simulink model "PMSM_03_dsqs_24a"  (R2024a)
settings: Solver=ode45  StartTime=0.0  StopTime=0.1  RelTol=1e-3  EnableMultiTasking=on
undefined symbols (not defined in the file): by, established, Flux, linkage, magnets, V
libraries: spsControlledVoltageSourceLib x3, spsCurrentMeasurementLib x3, spsPermanentMagnetSynchronousMachineLib x1, spspowerguiLib x1

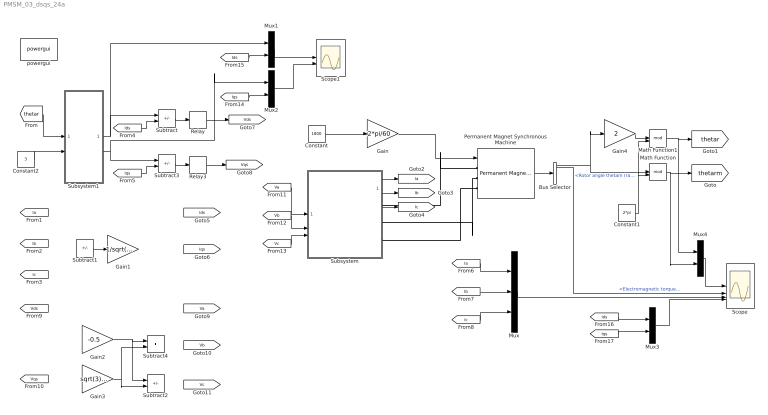
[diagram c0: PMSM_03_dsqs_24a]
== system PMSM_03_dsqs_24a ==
  Bus Selector : BusSelector  OutputSignals=Rotor angle thetam (rad),Electromagnetic torque Te (N*m)
  Constant : Constant  Value=1800
  Constant1 : Constant  Value=2*pi
  Constant2 : Constant  Value=3
  Gain : Gain  Gain=2*pi/60
  Gain1 : Gain  Gain=1/sqrt(3)
  Gain2 : Gain  Gain=-0.5
  Gain3 : Gain  Gain=sqrt(3)/2
  Gain4 : Gain  Gain=2
  Math Function : Math  Operator=mod  SignedPower=on
  Math Function1 : Math  Operator=mod  SignedPower=on
  Mux : Mux  Inputs=3
  Mux{1..4} (4 alike) : Mux  Inputs=2
  Permanent Magnet Synchronous Machine : spsPermanentMagnetSynchronousMachineLib/Permanent Magnet Synchronous Machine  NbPhases=3  FluxDistribution=Sinusoidal  RotorType=Round  MechanicalLoad=Speed w  PresetModel=No  ShowDetailedParameters=on  MeasurementBus=off  Resistance=0.423  Inductance=8.5e-3  dqInductances=[8.5e-3,8.5e-3]  La=0.00476  MachineConstant=Flux linkage established by magnets (V.s)  Flux=0.422  VoltageCst=153.0847  TorqueCst=1.266  Flat=120  Mechanical=[0.03 0.04 4 0]  PolePairs=2  InitialConditions=[0,0, 0,0]  InitialConditions5ph=[0 0 0 0 0 0]  RefAngle=Aligned with phase A axis (original Park)  IterativeDiscreteModel=Trapezoidal non iterative  TsBlock=-1  TsPowergui=0
  Relay : Relay  OnSwitchValue=0.2  OffSwitchValue=-0.2  OffOutputValue=-1
  Relay3 : Relay  OnSwitchValue=0.2  OffSwitchValue=-0.2  OffOutputValue=-1
  Scope : Scope  NumInputPorts=4
  Scope1 : Scope  NumInputPorts=2
  Subsystem : Subsystem
  Subsystem1 : Subsystem
  Subtract{,1..3} (4 alike) : Sum  Inputs=+-
  Subtract4 : Sum
  powergui : spspowerguiLib/powergui  Priority=1  SimulationMode=Continuous  SampleTime=50e-6  frequency=60  Iterations=50  frequencyindice=0  Pbase=100e6  ErrMax=1e-4  UnitsV=kV  UnitsW=MW  buscounter=0  FunctionMessages=off  echomessages=off  EnableUseOfTLC=off  CurrentSourceSwitches=off  DisableSnubberDevices=on  DisableRonSwitches=on  DisableVfSwitches=on  DisplayEquations=off  AutomaticDiscreteSolvers=off  SolverType=Tustin  Interpol=off  ExternalGateDelay=off  methode=off  Ts=0  x0status=blocks  SPID=on  SwTol=0  HookPort=off  NonlinearTolerance=1e-4  nMaxIteration=100  ContinueOnMaxIteration=off  RestoreLinks=warning  ResistiveCurrentMeasurement=off  Frange=[0:2:500]  Ylog=off  Xlog=on  ShowGrid=off  save=off  variable=ZData  structure=0  ZoomFFT=off  StartTime=0.0  cycles=1  DisplayStyle=1  fundamental=60  FreqAxis=off  MaxFrequency=1000  frequencyindicesteady=1  RmsSteady=1  display=off
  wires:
  Gain/1 -> Permanent Magnet Synchronous Machine/1
  Constant/1 -> Gain/1
  Subtract/1 -> Relay/1
  Permanent Magnet Synchronous Machine/1 -> Bus Selector/1
  Mux/1 -> Scope/3
  Bus Selector/2 -> Scope/2  "<Electromagnetic torque Te (N*m)>"
  Bus Selector/1 -> Gain4/1, Math Function/1  "<Rotor angle thetam (rad)>"
  Constant1/1 -> Math Function1/2, Math Function/2
  Math Function/1 -> Mux4/2, [thetarm]
  Gain4/1 -> Math Function1/1
  Math Function1/1 -> Mux4/1, [thetar]
  [thetar] -> Subsystem1/1(In1)
  Constant2/1 -> Subsystem1/2(In2)
  Subtract3/1 -> Relay3/1
  Subsystem1/1(Out1) -> Mux1/1, Subtract/1
  Subsystem1/2(Out2) -> Mux2/1, Subtract3/1
  Subsystem/1(Out1) -> [Ia]
  Subsystem/2(Out2) -> [Ib]
  Subsystem/3(Out3) -> [Ic]
  [Ids] -> Subtract/2
  [Iqs] -> Subtract3/2
  [Ia] -> Mux/1
  [Ib] -> Mux/2
  [Ic] -> Mux/3
  Relay/1 -> [Vds]
  Relay3/1 -> [Vqs]
  [Vc] -> Subsystem/3(In3)
  [Vb] -> Subsystem/2(In2)
  [Va] -> Subsystem/1(In1)
  Mux2/1 -> Scope1/2
  Mux1/1 -> Scope1/1
  [Ids] -> Mux1/2
  [Iqs] -> Mux2/2
  Mux3/1 -> Scope/4
  [Ids] -> Mux3/1
  [Iqs] -> Mux3/2
  Mux4/1 -> Scope/1
  Subtract1/1 -> Gain1/1
  Gain2/1 -> Subtract2/1, Subtract4/1
  Gain3/1 -> Subtract2/2, Subtract4/2
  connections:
  Subsystem/RConn1 -- Permanent Magnet Synchronous Machine/LConn1
  Permanent Magnet Synchronous Machine/LConn2 -- Subsystem/RConn2
  Subsystem/RConn3 -- Permanent Magnet Synchronous Machine/LConn3

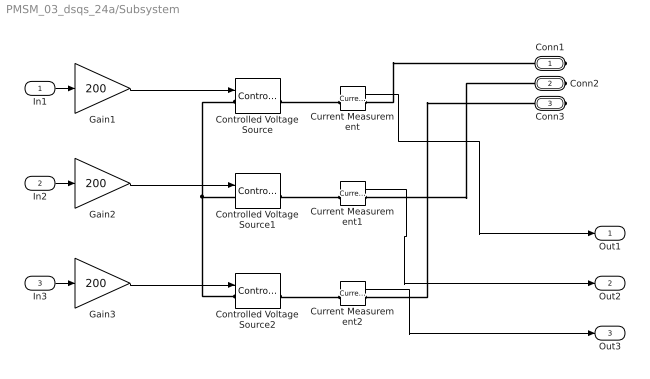
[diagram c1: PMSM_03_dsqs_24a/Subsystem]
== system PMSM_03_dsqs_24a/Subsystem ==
  In1 : Inport
  In2 : Inport  Port=2
  In3 : Inport  Port=3
  Controlled Voltage Source : spsControlledVoltageSourceLib/Controlled Voltage Source  Initialize=on  Source_Type=AC  Amplitude=0  Phase=0  Frequency=0  Measurements=None
  Controlled Voltage Source1 : spsControlledVoltageSourceLib/Controlled Voltage Source  Initialize=on  Source_Type=AC  Amplitude=0  Phase=0  Frequency=0  Measurements=None
  Controlled Voltage Source2 : spsControlledVoltageSourceLib/Controlled Voltage Source  Initialize=on  Source_Type=AC  Amplitude=0  Phase=0  Frequency=0  Measurements=None
  Current Measurement : spsCurrentMeasurementLib/Current Measurement  PhasorSimulation=off  OutputType=Complex  PSBequivalent=0
  Current Measurement1 : spsCurrentMeasurementLib/Current Measurement  PhasorSimulation=off  OutputType=Complex  PSBequivalent=0
  Current Measurement2 : spsCurrentMeasurementLib/Current Measurement  PhasorSimulation=off  OutputType=Complex  PSBequivalent=0
  Gain1 : Gain  Gain=200
  Gain2 : Gain  Gain=200
  Gain3 : Gain  Gain=200
  Conn1 : PMIOPort  Side=Right
  Conn2 : PMIOPort  Port=2  Side=Right
  Conn3 : PMIOPort  Port=3  Side=Right
  Out1 : Outport
  Out2 : Outport  Port=2
  Out3 : Outport  Port=3
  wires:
  In1/1 -> Gain1/1
  In2/1 -> Gain2/1
  In3/1 -> Gain3/1
  Current Measurement1/1 -> Out2/1
  Gain3/1 -> Controlled Voltage Source2/1
  Gain2/1 -> Controlled Voltage Source1/1
  Gain1/1 -> Controlled Voltage Source/1
  Current Measurement2/1 -> Out3/1
  Current Measurement/1 -> Out1/1
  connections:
  Current Measurement/RConn1 -- Conn1/RConn1
  Controlled Voltage Source/LConn1 -- Controlled Voltage Source1/LConn1 -- Controlled Voltage Source2/LConn1
  Controlled Voltage Source/RConn1 -- Current Measurement/LConn1
  Conn2/RConn1 -- Current Measurement1/RConn1
  Current Measurement2/RConn1 -- Conn3/RConn1
  Controlled Voltage Source1/RConn1 -- Current Measurement1/LConn1
  Controlled Voltage Source2/RConn1 -- Current Measurement2/LConn1

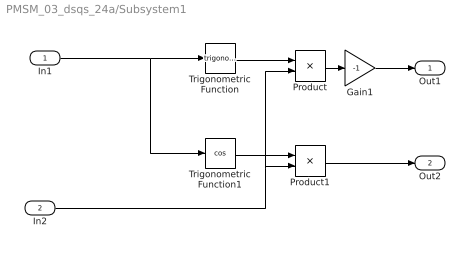
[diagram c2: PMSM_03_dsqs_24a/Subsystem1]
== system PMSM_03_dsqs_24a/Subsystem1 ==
  In1 : Inport
  In2 : Inport  Port=2
  Gain1 : Gain  Gain=-1
  Product : Product
  Product1 : Product
  Trigonometric Function : Trigonometry
  Trigonometric Function1 : Trigonometry  Operator=cos
  Out1 : Outport
  Out2 : Outport  Port=2
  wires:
  Trigonometric Function1/1 -> Product1/1
  Product/1 -> Gain1/1
  Product1/1 -> Out2/1
  In1/1 -> Trigonometric Function1/1, Trigonometric Function/1
  Trigonometric Function/1 -> Product/1
  Gain1/1 -> Out1/1
  In2/1 -> Product/2, Product1/2
